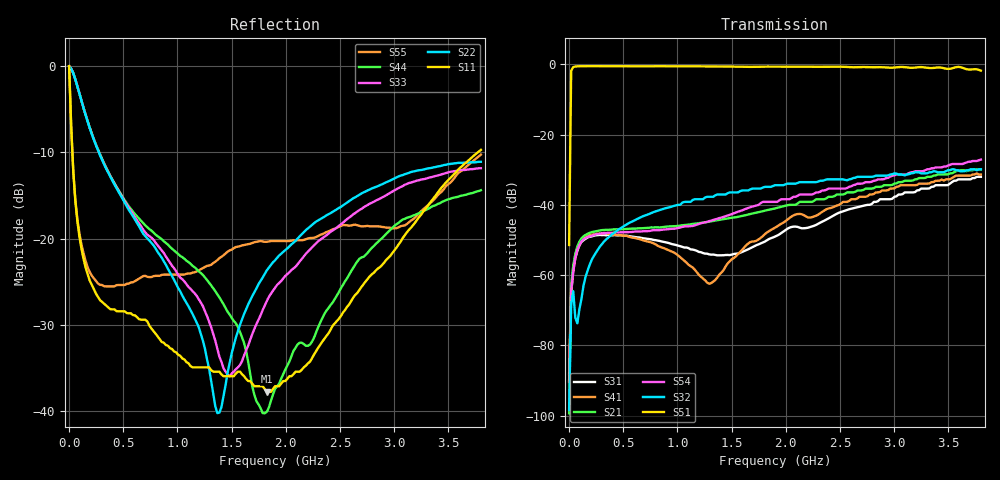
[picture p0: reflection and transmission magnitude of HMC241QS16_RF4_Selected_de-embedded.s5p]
! Hittite Microwave Corporation
! 20 Alpha Road
! Chelmsford, MA 01824
! Tel: 978-250-3343
! Fax: 978-250-3373
! Device: HMC241QS16, DC-3.5 GHz GaAs MMIC SP4T Non-Reflective Switch in 16 lead QSOP package
! Misc: Data was de-embedded to package pins.
!  Port 1 = RFC
!  Port 2 = RF1
!  Port 3 = RF2
!  Port 4 = RF3
!  Port 5 = RF4
!  Vdd  = + 5 V
!  RF4 selected, Vctl= 0/+5 V
!  Data reformated to new Touchstone file format - Tue Jan 09 10:11:19 2007
# MHz S DB R 50
! 5 Port Network Data
! freq  dbS11  angS11  dbS12  angS12  dbS13  angS13  dbS14  angS14
!  dbS15  angS15
!  dbS21  angS21  dbS22  angS22  dbS23  angS23
!  dbS24  angS24  dbS25  angS25
!  dbS31  angS31  dbS32  angS32
!  dbS33  angS33  dbS34  angS34  dbS35  angS35
!  dbS41  angS41
!  dbS42  angS42  dbS43  angS43  dbS44  angS44  dbS45  angS45
!  dbS51  angS51  dbS52  angS52  dbS53  angS53  dbS54  angS54
!  dbS55  angS55
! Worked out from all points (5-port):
!   201 points, 30 kHz to 3.8 GHz, reference 50 ohm
!   strongest paths, dB at 30 kHz, 950 MHz, 1.9 GHz, 2.85 GHz, 3.8 GHz:
!     S51: -51.4, -0.6, -0.7, -0.8, -1.8
!     S32: -98.4, -40.5, -34.4, -31.7, -29.9
!     S54: -90.5, -46.8, -39.2, -32.8, -27.1
!     S21: -99.3, -46.1, -41.0, -34.9, -29.9
!     S41: -88.2, -53.3, -46.5, -36.5, -31.4
!     S31: -90.1, -51.2, -49.1, -39.0, -32.0
!   lowest |S11| = -37.7 dB at 1.824 GHz (marker M1), VSWR 1.03, Z = 49.1 - j0.962 ohm
!   |S11| at or under -10 dB: 30.27 MHz to 3.771 GHz (3.74 GHz wide, 197 % of centre)
